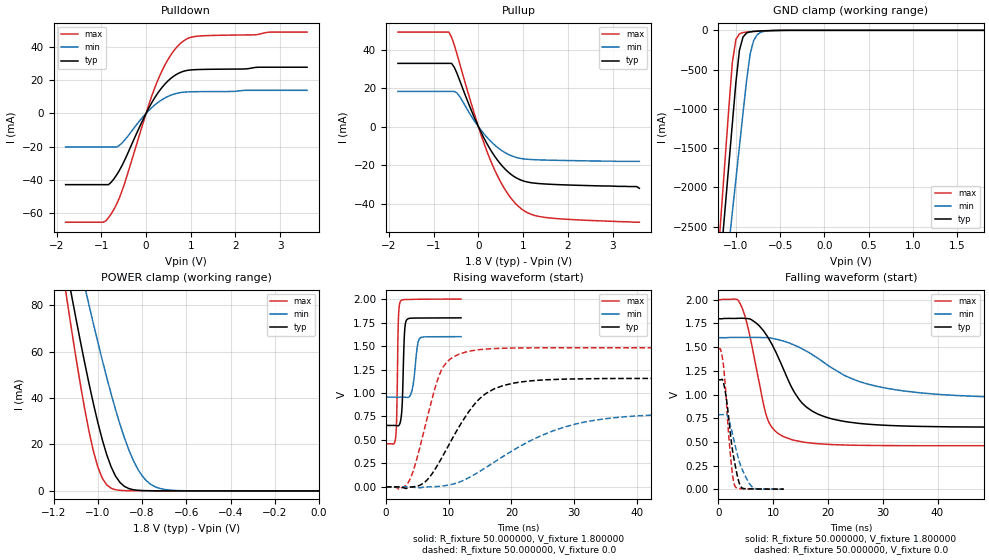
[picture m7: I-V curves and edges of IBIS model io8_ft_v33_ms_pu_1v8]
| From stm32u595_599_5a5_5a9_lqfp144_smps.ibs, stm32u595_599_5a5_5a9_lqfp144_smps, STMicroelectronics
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|   Model io8_ft_v33_ms_pu_1v8
[Model]  io8_ft_v33_ms_pu_1v8
Model_type I/O
Polarity   Non-Inverting
Enable   Active-Low
Vinl =   0.540000V
Vinh =   1.260000V
Vmeas =  0.900000V
Cref =   50.000000pF
Rref =   100.000000M
Vref =   0.0V
C_comp   3.087500pF   3.086600pF   3.135700pF
[Temperature Range]   25.000000   0.140000k   -40.000000
[Pullup Reference]   1.800000V   1.600000V   2.000000V
[Pulldown Reference]   0.0V   0.0V   0.0V
[POWER Clamp Reference]   1.800000V   1.600000V   2.000000V
[GND Clamp Reference]   0.0V   0.0V   0.0V
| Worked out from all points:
|   slope of the pulldown table from 0 to 0.27 V, typ, clamps not added: 21.7 ohm
|   slope of the pullup table from 0 to 0.27 V, typ, clamps not added: 22.6 ohm
|   GND clamp passes 1 mA (typ) near -0.51 V on its own axis
|   POWER clamp passes 1 mA (typ) near -0.86 V on its own axis
|   rising waveform, R_fixture 50.000000, V_fixture 1.800000: 20-80 % time 315ps typ, 627ps min, 225ps max; typ from 0.655 V to 1.8 V
|   rising waveform, R_fixture 50.000000, V_fixture 0.0: 20-80 % time 6.48ns typ, 13.4ns min, 3.57ns max; typ from 0.001 V to 1.16 V
|   falling waveform, R_fixture 50.000000, V_fixture 1.800000: 20-80 % time 6.38ns typ, 13.4ns min, 3.35ns max; typ from 1.8 V to 0.655 V
|   falling waveform, R_fixture 50.000000, V_fixture 0.0: 20-80 % time 1.6ns typ, 2.38ns min, 1.18ns max; typ from 1.16 V to 0.001 V
[Pulldown]
|Voltage   I(typ)   I(min)   I(max)
-1.8V     -42.74mA   -20.21mA   -65.25mA
-960mV    -42.74mA   -20.21mA   -65.25mA
-780mV    -41.3mA    -20.21mA   -60.25mA
-660mV    -37mA      -20.2mA    -54.5mA
-540mV    -31.39mA   -17.82mA   -46.65mA
0V        0A         0A         0A
240mV     11.28mA    6.002mA    18.38mA
480mV     19.17mA    10.02mA    31.83mA
780mV     24.67mA    12.5mA     42.21mA
960mV     25.9mA     12.9mA     45.21mA
1.2V      26.29mA    13.01mA    46.37mA
3.6V      27.66mA    13.81mA    48.71mA
[Pullup]
|Voltage   I(typ)   I(min)   I(max)
-1.8V     32.87mA    18.3mA     49.12mA
-660mV    32.87mA    18.3mA     49.12mA
-600mV    32.87mA    18.3mA     46.4mA
-480mV    27.73mA    17.56mA    37.8mA
-60mV     3.108mA    1.975mA    4.436mA
240mV     -10.82mA   -6.752mA   -15.73mA
420mV     -17.18mA   -10.64mA   -25.23mA
600mV     -22.1mA    -13.54mA   -32.82mA
960mV     -27.82mA   -16.55mA   -42.66mA
1.2V      -29.16mA   -17.09mA   -45.68mA
1.56V     -29.85mA   -17.37mA   -47.3mA
3.6V      -32mA      -18mA      -49.6mA
[GND_clamp]
|Voltage   I(typ)   I(min)   I(max)
-1.8V     -9.707A    -9.942A    -9.774A
-1.2V     -3.309A    -4.006A    -2.864A
-1.16V    -2.777A    -3.584A    -2.239A
-1.12V    -2.246A    -3.162A    -1.614A
-1.04V    -1.186A    -2.319A    -408.6mA
-1V       -663.9mA   -1.898A    -117.8mA
-960mV    -254mA     -1.478A    -45.14mA
-920mV    -86.03mA   -1.06A     -28.58mA
-840mV    -19.12mA   -308.9mA   -18.74mA
-800mV    -13.39mA   -130.8mA   -15.31mA
-720mV    -7.948mA   -25.37mA   -9.381mA
1.8V      0A         14.97nA    0A
[POWER_clamp]
|Voltage   I(typ)   I(min)   I(max)
-1.8V     470.9mA    433.7mA    554.6mA
-1.14V    95.29mA    122.7mA    82.89mA
-1.12V    85mA       114mA      70.34mA
-1.06V    55.55mA    88.43mA    35.74mA
-1.04V    46.38mA    80.17mA    25.83mA
-1V       29.54mA    64.14mA    10.37mA
-940mV    10.43mA    41.88mA    1.179mA
-900mV    3.662mA    28.79mA    252.8uA
-840mV    528.6uA    13.26mA    97.33uA
-800mV    159uA      6.55mA     88.9uA
-740mV    60.12uA    1.751mA    70.99uA
0V        0A         18.15nA    0A
[Ramp]
| variable   typ   min   max
dV/dt_r  0.69287/6.47442n   0.47194/13.35312n   0.88855/3.56621n
dV/dt_f  0.68715/6.37121n   0.38558/13.39721n   0.92439/3.34998n
R_load = 50.000000
[Rising Waveform]
R_fixture= 50.000000
V_fixture= 1.800000
V_fixture_min= 1.600000
V_fixture_max= 2.000000
|time   V(typ)   V(min)   V(max)
0s        654.8mV    956mV      459.4mV
1.586ns   654.1mV    956.1mV    542.7mV
1.73ns    653mV      956.1mV    761.2mV
1.994ns   651.8mV    956.1mV    1.779V
2.33ns    699mV      956mV      1.977V
2.619ns   902.5mV    955.8mV    1.991V
2.979ns   1.648V     954.7mV    1.995V
3.315ns   1.778V     952.3mV    1.995V
5.405ns   1.798V     1.583V     1.998V
11.96ns   1.8V       1.6V       2V
[Rising Waveform]
R_fixture= 50.000000
V_fixture= 0.0
V_fixture_min= 0.0
V_fixture_max= 0.0
|time   V(typ)   V(min)   V(max)
0s        615.9uV    687.1uV    590.9uV
3.524ns   -8.395mV   297.1uV    43.55mV
6.246ns   53.74mV    -903.4uV   644.2mV
8.809ns   298.9mV    7.745mV    1.239V
12.97ns   778.8mV    90.35mV    1.441V
15.86ns   991.1mV    203.4mV    1.467V
18.74ns   1.08V      327.5mV    1.476V
26.75ns   1.144V     599.6mV    1.481V
33.79ns   1.153V     715.4mV    1.481V
79.76ns   1.155V     787.4mV    1.481V
[Falling Waveform]
R_fixture= 50.000000
V_fixture= 1.800000
V_fixture_min= 1.600000
V_fixture_max= 2.000000
|time   V(typ)   V(min)   V(max)
0s        1.8V       1.6V       2V
4.004ns   1.805V     1.603V     1.959V
5.445ns   1.801V     1.603V     1.703V
8.969ns   1.613V     1.6V       746.1mV
10.57ns   1.441V     1.584V     605.5mV
13.45ns   1.069V     1.532V     522.9mV
18.9ns    776.4mV    1.354V     477.7mV
24.66ns   702.5mV    1.16V      464.4mV
33.63ns   667.9mV    1.039V     460.2mV
79.76ns   654.8mV    956mV      459.4mV
[Falling Waveform]
R_fixture= 50.000000
V_fixture= 0.0
V_fixture_min= 0.0
V_fixture_max= 0.0
|time   V(typ)   V(min)   V(max)
0s        1.155V     787.4mV    1.481V
432.4ps   1.155V     787.4mV    1.475V
961ps     1.124V     787.3mV    1.306V
1.586ns   917.8mV    787.4mV    845.8mV
2.282ns   558.9mV    661.8mV    330.3mV
2.715ns   372.6mV    556mV      111.1mV
3.051ns   267.9mV    472.3mV    31.89mV
4.06ns    33.43mV    254.6mV    6.31mV
6.126ns   3.343mV    27.88mV    1.839mV
11.96ns   615.9uV    687.1uV    590.9uV
